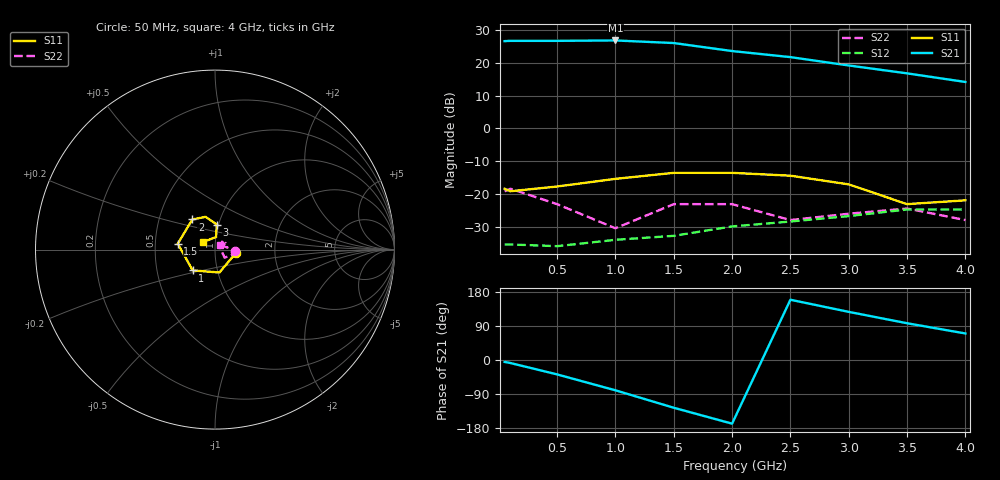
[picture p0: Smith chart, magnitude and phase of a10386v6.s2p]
!  INA-10386  S PARAMETERS
!  Vd = 6 V  LAST UPDATED 06-23-94
# ghz s ma r 50
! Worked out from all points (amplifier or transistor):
!   10 points, 50 MHz to 4 GHz, reference 50 ohm
!   highest |S21| = 26.8 dB at 1 GHz (marker M1)
!   |S21| within 3 dB of that: start of sweep to 1.953 GHz
!   unconditionally stable (mu >= 1): start of sweep to end of sweep
!   at 100 MHz: K = 1.50, MAG = 26.9 dB, |S12| = -35.4 dB
!   at 2 GHz: K = 1.23, MAG = 23.8 dB, |S12| = -29.9 dB
!   at 4 GHz: K = 1.82, MAG = 14.2 dB, |S12| = -24.7 dB
!   S11 on the Smith chart (normalised r, x): 50 MHz: 1.27, -0.05; 1 GHz: 0.76, -0.18; 1.5 GHz: 0.66, +0.05; 2 GHz: 0.74, +0.26; 3 GHz: 0.98, +0.28; 4 GHz: 0.87, +0.07
0.05  0.12 -9.0  21.4 -5.0  0.017 1.0  0.11 -3.0
0.1  0.11 -17.0  21.6 -8.0  0.017 3.0  0.12 -10.0
0.5  0.13 -79.0  21.6 -38.0  0.016 10.0  0.07 -40.0
1  0.17 -137.0  21.9 -80.0  0.02 43.0  0.03 18.0
1.5  0.21 171.0  20 -126.0  0.023 53.0  0.07 32.0
2  0.21 127.0  15.1 -168.0  0.032 55.0  0.07 9.0
2.5  0.19 106.0  12.2 159.0  0.038 58.0  0.04 42.0
3  0.14 86.0  9.1 127.0  0.046 55.0  0.05 56.0
3.5  0.07 85.0  6.9 97.0  0.058 50.0  0.06 47.0
4  0.08 148.0  5.1 70.0  0.058 51.0  0.04 40.0
